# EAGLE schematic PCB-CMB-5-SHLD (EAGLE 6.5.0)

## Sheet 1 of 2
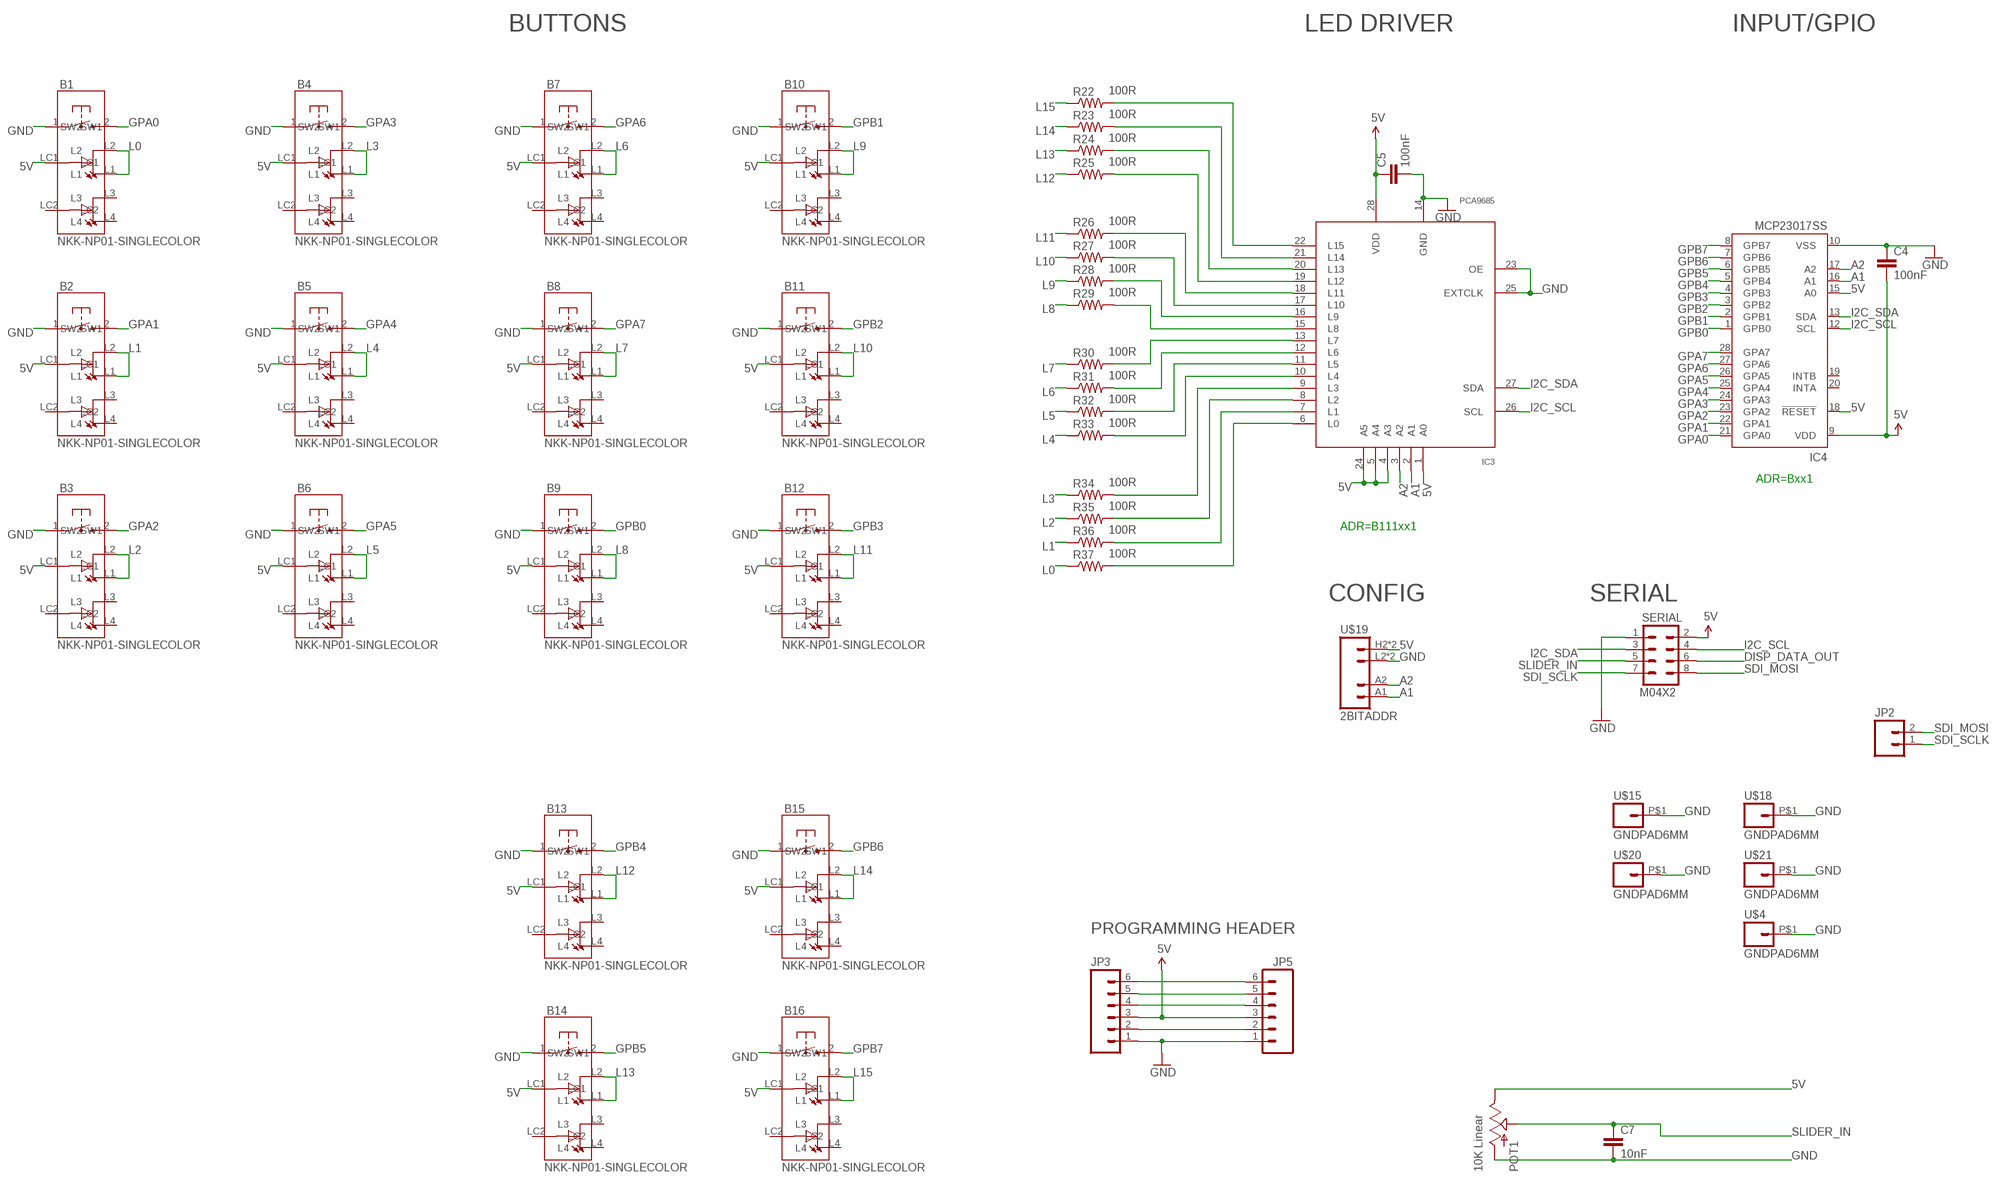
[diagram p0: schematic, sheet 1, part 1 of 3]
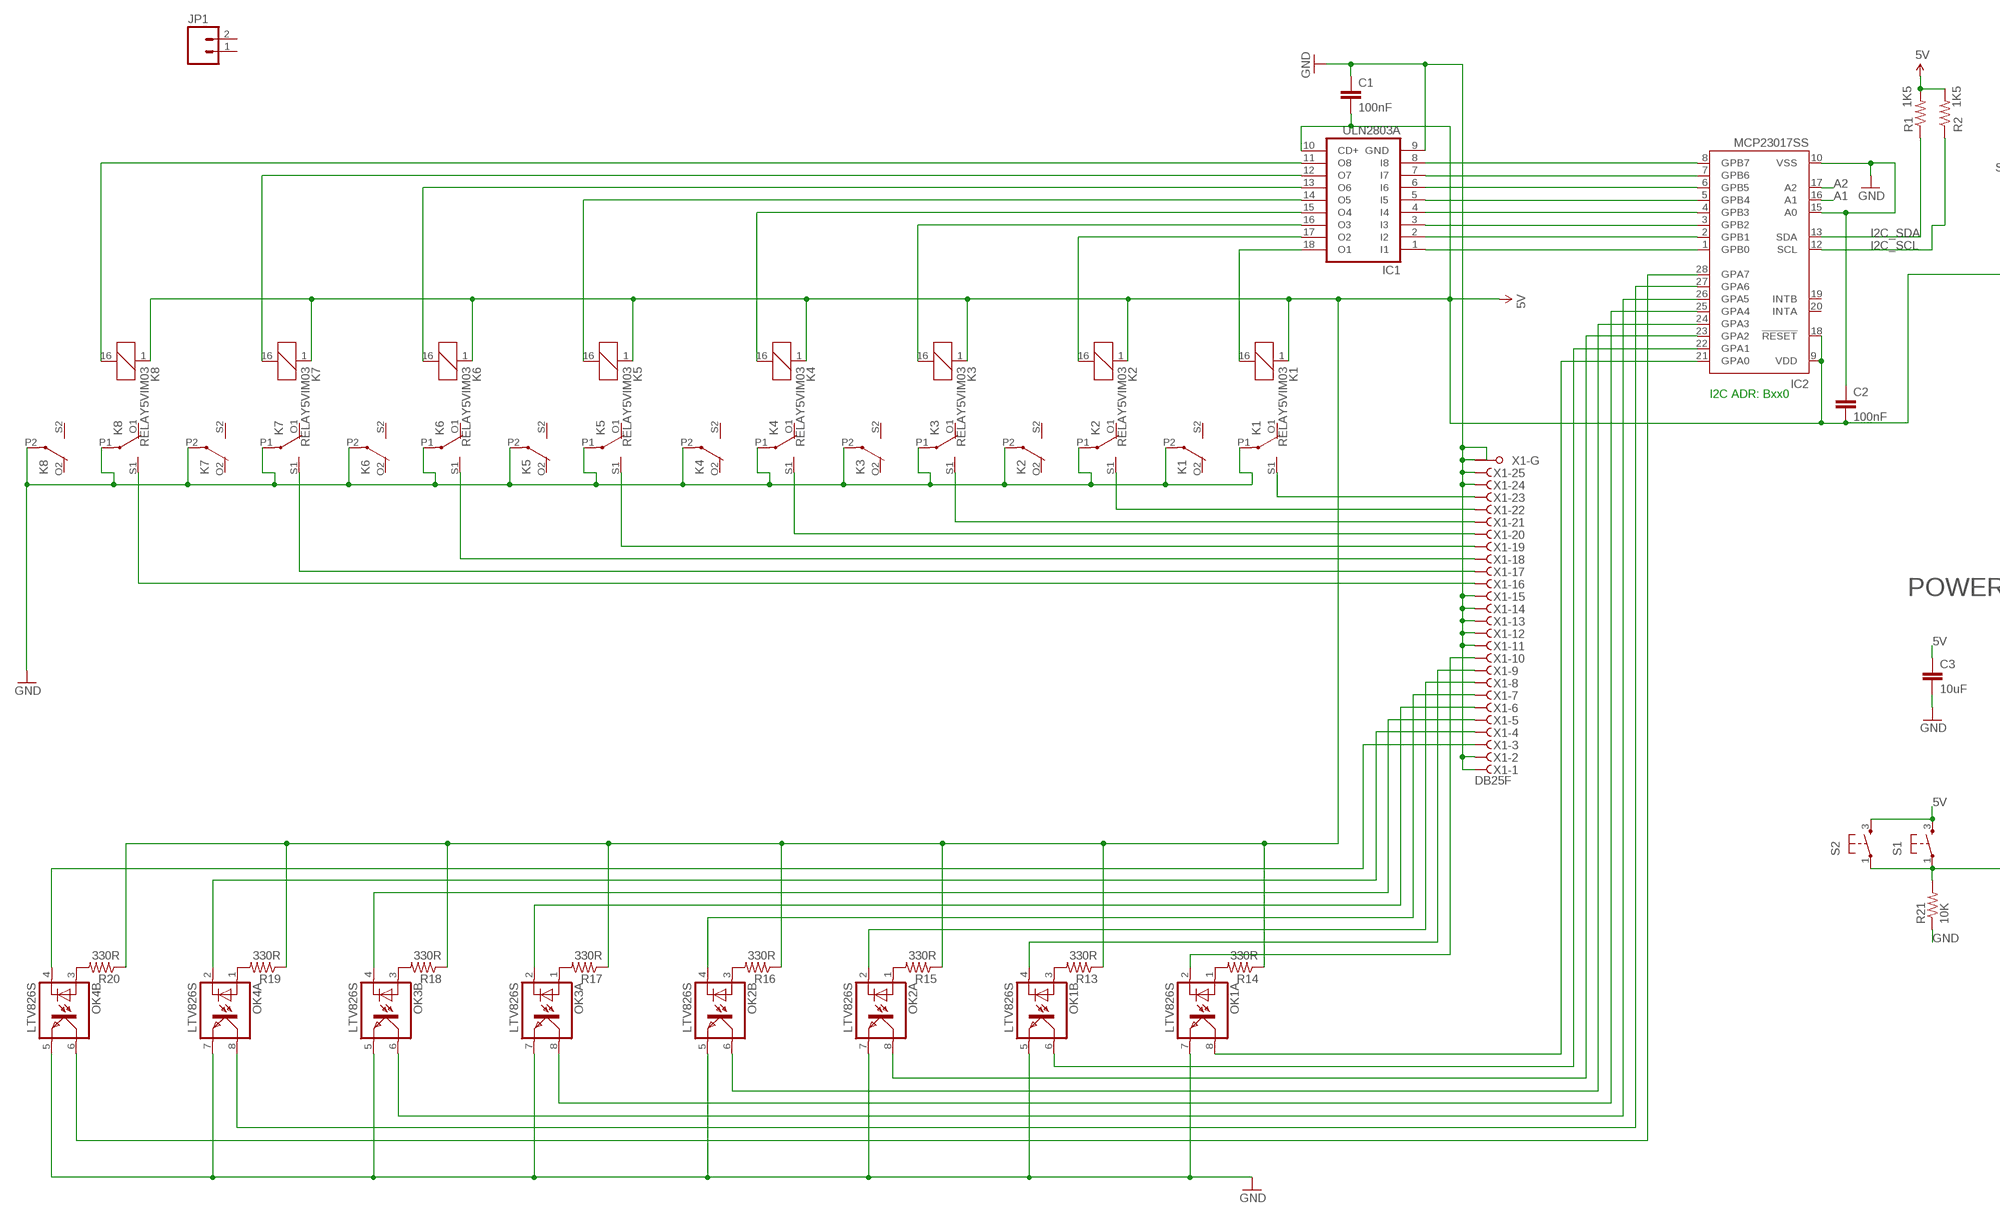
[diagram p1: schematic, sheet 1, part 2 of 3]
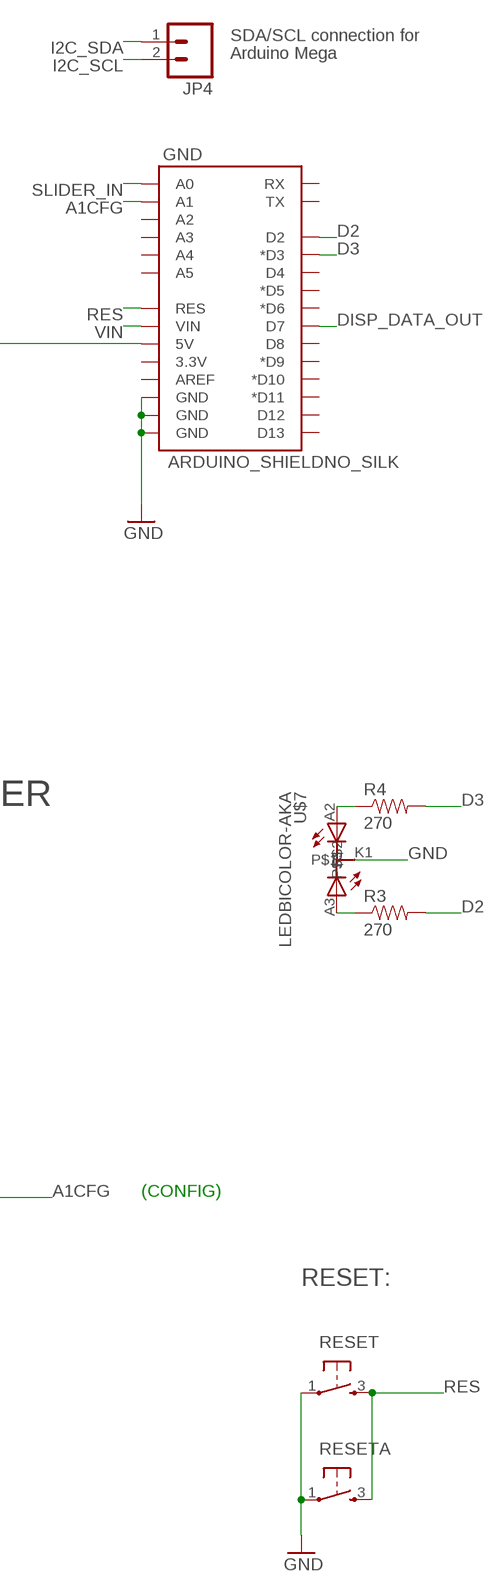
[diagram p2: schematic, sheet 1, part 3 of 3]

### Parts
B1  NKK-NP01-SINGLECOLOR  [NKK-NP01]
B2  NKK-NP01-SINGLECOLOR  [NKK-NP01]
B3  NKK-NP01-SINGLECOLOR  [NKK-NP01]
B4  NKK-NP01-SINGLECOLOR  [NKK-NP01]
B5  NKK-NP01-SINGLECOLOR  [NKK-NP01]
B6  NKK-NP01-SINGLECOLOR  [NKK-NP01]
B7  NKK-NP01-SINGLECOLOR  [NKK-NP01]
B8  NKK-NP01-SINGLECOLOR  [NKK-NP01]
B9  NKK-NP01-SINGLECOLOR  [NKK-NP01]
B10  NKK-NP01-SINGLECOLOR  [NKK-NP01]
B11  NKK-NP01-SINGLECOLOR  [NKK-NP01]
B12  NKK-NP01-SINGLECOLOR  [NKK-NP01]
B13  NKK-NP01-SINGLECOLOR  [NKK-NP01]
B14  NKK-NP01-SINGLECOLOR  [NKK-NP01]
B15  NKK-NP01-SINGLECOLOR  [NKK-NP01]
B16  NKK-NP01-SINGLECOLOR  [NKK-NP01]
C1  100nF  CAP0805  [0805]
C2  100nF  CAP0603-CAP  [0603-CAP]
C3  10uF  CAP0805  [0805]
C4  100nF  CAP0603-CAP  [0603-CAP]
C5  100nF  CAP0603-CAP  [0603-CAP]
C7  10nF  CAP0603-CAP  [0603-CAP]
GND  ARDUINO_SHIELDNO_SILK  [DUEMILANOVE_VIAS]
IC1  ULN2803A  ULN2803ASO18W  [SO18W]
IC2  MCP23017SS  [SSOP28]
IC3  PCA9685  [TSSOP28]
IC4  MCP23017SS  [SSOP28]
JP1  M02PTH  [1X02]
JP2  M02PTH  [1X02]
JP3  M06POLAR  [MOLEX-1X6]
JP4  M02PTH  [1X02]
JP5  M06POLAR  [MOLEX-1X6]
K1  RELAY5VIM03  [DS2Y]
K2  RELAY5VIM03  [DS2Y]
K3  RELAY5VIM03  [DS2Y]
K4  RELAY5VIM03  [DS2Y]
K5  RELAY5VIM03  [DS2Y]
K6  RELAY5VIM03  [DS2Y]
K7  RELAY5VIM03  [DS2Y]
K8  RELAY5VIM03  [DS2Y]
OK1  LTV826S  [DIL8-SMD]
OK2  LTV826S  [DIL8-SMD]
OK3  LTV826S  [DIL8-SMD]
OK4  LTV826S  [DIL8-SMD]
POT1  10K Linear  SLIDER20  [SLIDER20]
R1  1K5  RESISTOR0603-RES  [0603-RES]
R2  1K5  RESISTOR0603-RES  [0603-RES]
R3  270  RESISTOR0603-RES  [0603-RES]
R4  270  RESISTOR0603-RES  [0603-RES]
R13  330R  RESISTOR0603-RES  [0603-RES]
R14  330R  RESISTOR0603-RES  [0603-RES]
R15  330R  RESISTOR0603-RES  [0603-RES]
R16  330R  RESISTOR0603-RES  [0603-RES]
R17  330R  RESISTOR0603-RES  [0603-RES]
R18  330R  RESISTOR0603-RES  [0603-RES]
R19  330R  RESISTOR0603-RES  [0603-RES]
R20  330R  RESISTOR0603-RES  [0603-RES]
R21  10K  RESISTOR0603-RES  [0603-RES]
R22  100R  RESISTOR0603-RES  [0603-RES]
R23  100R  RESISTOR0603-RES  [0603-RES]
R24  100R  RESISTOR0603-RES  [0603-RES]
R25  100R  RESISTOR0603-RES  [0603-RES]
R26  100R  RESISTOR0603-RES  [0603-RES]
R27  100R  RESISTOR0603-RES  [0603-RES]
R28  100R  RESISTOR0603-RES  [0603-RES]
R29  100R  RESISTOR0603-RES  [0603-RES]
R30  100R  RESISTOR0603-RES  [0603-RES]
R31  100R  RESISTOR0603-RES  [0603-RES]
R32  100R  RESISTOR0603-RES  [0603-RES]
R33  100R  RESISTOR0603-RES  [0603-RES]
R34  100R  RESISTOR0603-RES  [0603-RES]
R35  100R  RESISTOR0603-RES  [0603-RES]
R36  100R  RESISTOR0603-RES  [0603-RES]
R37  100R  RESISTOR0603-RES  [0603-RES]
RESET  TAC_SWITCH  [PUSHBUTTON]
RESETA  TAC_SWITCH  [PUSHBUTTON]
S1  TAC_SWITCH  [PUSHBUTTON]
S2  TAC_SWITCH  [PUSHBUTTON]
SERIAL  M04X2  [2X4]
U$4  GNDPAD6MM  [3.2MMPAD6MM]
U$7  LEDBICOLOR-AKA  [LED5MM-BICOLOR]
U$15  GNDPAD6MM  [3.2MMPAD6MM]
U$18  GNDPAD6MM  [3.2MMPAD6MM]
U$19  2BITADDR  [2BITADDR]
U$20  GNDPAD6MM  [3.2MMPAD6MM]
U$21  GNDPAD6MM  [3.2MMPAD6MM]
X1  DB25F  F25HPS  [F25HP]

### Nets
5V [PWR]: B1.LC1 B2.LC1 B3.LC1 B4.LC1 B5.LC1 B6.LC1 B7.LC1 B8.LC1 B9.LC1 B10.LC1 B11.LC1 B12.LC1 B13.LC1 B14.LC1 B15.LC1 B16.LC1 C1.2 C2.2 C3.1 C4.2 C5.1 GND.5V IC1.10(CD+) IC2.9(VDD) IC2.18(!RESET) IC3.1(A0) IC3.4(A3) IC3.5(A4) IC3.24(A5) IC3.28(VDD) IC4.9(VDD) IC4.15(A0) IC4.18(!RESET) JP3.3 JP5.3 K1.1 K2.1 K3.1 K4.1 K5.1 K6.1 K7.1 K8.1 POT1.1(E) R1.2 R2.2 R13.1 R14.1 R15.1 R16.1 R17.1 R18.1 R19.1 R20.1 S1.3 S2.3 SERIAL.2 U$19.H2(VCC) U$19.H3(VCC)
A1: IC2.16(A1) IC3.2(A1) IC4.16(A1) U$19.A1
A1CFG: GND.A1 R21.2 S1.1 S2.1
A2: IC2.17(A2) IC3.3(A2) IC4.17(A2) U$19.A2
D2: GND.D2 R3.2
D3: GND.D3(*D3) R4.2
DISP_DATA_OUT: GND.D7 SERIAL.6
GND [PWR]: B1.1(SW1) B2.1(SW1) B3.1(SW1) B4.1(SW1) B5.1(SW1) B6.1(SW1) B7.1(SW1) B8.1(SW1) B9.1(SW1) B10.1(SW1) B11.1(SW1) B12.1(SW1) B13.1(SW1) B14.1(SW1) B15.1(SW1) B16.1(SW1) C1.1 C2.1 C3.2 C4.1 C5.2 C7.2 GND.GND@0(GND) GND.GND@1(GND) GND.GND@2(GND) IC1.9(GND) IC2.10(VSS) IC2.15(A0) IC3.14(GND) IC3.23(OE) IC3.25(EXTCLK) IC4.10(VSS) JP3.1 JP5.1 K1.P1(2:P) K1.P2(3:P) K2.P1(2:P) K2.P2(3:P) K3.P1(2:P) K3.P2(3:P) K4.P1(2:P) K4.P2(3:P) K5.P1(2:P) K5.P2(3:P) K6.P1(2:P) K6.P2(3:P) K7.P1(2:P) K7.P2(3:P) K8.P1(2:P) K8.P2(3:P) OK1.5(B:EMIT) OK1.7(A:EMIT) OK2.5(B:EMIT) OK2.7(A:EMIT) OK3.5(B:EMIT) OK3.7(A:EMIT) OK4.5(B:EMIT) OK4.7(A:EMIT) POT1.3(A) R21.1 RESET.1 RESETA.1 SERIAL.1 U$4.P$1 U$7.K1 U$15.P$1 U$18.P$1 U$19.L2(GND) U$19.L3(GND) U$20.P$1 U$21.P$1 X1.1(-1:F) X1.2(-2:F) X1.11(-11:F) X1.12(-12:F) X1.13(-13:F) X1.14(-14:F) X1.15(-15:F) X1.24(-24:F) X1.25(-25:F) X1.G1(-G:G1) X1.G2(-G:G2)
GPA0: B1.2(SW2) IC4.21(GPA0)
GPA1: B2.2(SW2) IC4.22(GPA1)
GPA2: B3.2(SW2) IC4.23(GPA2)
GPA3: B4.2(SW2) IC4.24(GPA3)
GPA4: B5.2(SW2) IC4.25(GPA4)
GPA5: B6.2(SW2) IC4.26(GPA5)
GPA6: B7.2(SW2) IC4.27(GPA6)
GPA7: B8.2(SW2) IC4.28(GPA7)
GPB0 [PWR]: B9.2(SW2) IC4.1(GPB0)
GPB1: B10.2(SW2) IC4.2(GPB1)
GPB2: B11.2(SW2) IC4.3(GPB2)
GPB3: B12.2(SW2) IC4.4(GPB3)
GPB4: B13.2(SW2) IC4.5(GPB4)
GPB5: B14.2(SW2) IC4.6(GPB5)
GPB6: B15.2(SW2) IC4.7(GPB6)
GPB7: B16.2(SW2) IC4.8(GPB7)
I2C_SCL: IC2.12(SCL) IC3.26(SCL) IC4.12(SCL) JP4.2 R2.1 SERIAL.4
I2C_SDA: IC2.13(SDA) IC3.27(SDA) IC4.13(SDA) JP4.1 R1.1 SERIAL.3
L0: B1.L1 B1.L2 R37.1
L1: B2.L1 B2.L2 R36.1
L2: B3.L1 B3.L2 R35.1
L3: B4.L1 B4.L2 R34.1
L4: B5.L1 B5.L2 R33.1
L5: B6.L1 B6.L2 R32.1
L6: B7.L1 B7.L2 R31.1
L7: B8.L1 B8.L2 R30.1
L8: B9.L1 B9.L2 R29.1
L9: B10.L1 B10.L2 R28.1
L10: B11.L1 B11.L2 R27.1
L11: B12.L1 B12.L2 R26.1
L12: B13.L1 B13.L2 R25.1
L13: B14.L1 B14.L2 R24.1
L14: B15.L1 B15.L2 R23.1
L15: B16.L1 B16.L2 R22.1
N$1 [RELAY LINES]: K1.S1(2:S) X1.23(-23:F)
N$2: IC3.13(L7) R30.2
N$3: JP3.4 JP5.4
N$4: IC1.18(O1) K1.16
N$5: IC1.1(I1) IC2.1(GPB0)
N$6 [RELAY LINES]: K2.S1(2:S) X1.22(-22:F)
N$7: R4.1 U$7.A2
N$8: JP3.5 JP5.5
N$9: IC1.17(O2) K2.16
N$10 [RELAY LINES]: K3.S1(2:S) X1.21(-21:F)
N$11: R3.1 U$7.A3
N$12: JP3.2 JP5.2
N$13: IC1.16(O3) K3.16
N$14 [RELAY LINES]: K4.S1(2:S) X1.20(-20:F)
N$17: IC1.15(O4) K4.16
N$18 [RELAY LINES]: K5.S1(2:S) X1.19(-19:F)
N$19: IC3.12(L6) R31.2
N$21: IC1.14(O5) K5.16
N$22 [RELAY LINES]: K6.S1(2:S) X1.18(-18:F)
N$23: IC3.11(L5) R32.2
N$25: IC1.13(O6) K6.16
N$26 [RELAY LINES]: K7.S1(2:S) X1.17(-17:F)
N$29: IC1.12(O7) K7.16
N$30 [RELAY LINES]: K8.S1(2:S) X1.16(-16:F)
N$31: IC3.10(L4) R33.2
N$33: IC1.11(O8) K8.16
N$34: IC1.2(I2) IC2.2(GPB1)
N$35: IC1.3(I3) IC2.3(GPB2)
N$36: IC1.4(I4) IC2.4(GPB3)
N$37: IC1.5(I5) IC2.5(GPB4)
N$38: IC1.6(I6) IC2.6(GPB5)
N$39: IC1.7(I7) IC2.7(GPB6)
N$40: IC1.8(I8) IC2.8(GPB7)
N$45: JP3.6 JP5.6
N$47: OK1.3(B:A) R13.2
N$48: OK1.1(A:A) R14.2
N$49 [INput lines]: OK1.2(A:C) X1.10(-10:F)
N$50: OK2.1(A:A) R15.2
N$51: IC2.21(GPA0) OK1.8(A:COL)
N$52: OK2.3(B:A) R16.2
N$53: OK3.1(A:A) R17.2
N$54: OK3.3(B:A) R18.2
N$55 [INput lines]: OK3.2(A:C) X1.6(-6:F)
N$56: OK4.1(A:A) R19.2
N$57: OK4.3(B:A) R20.2
N$58: IC3.9(L3) R34.2
N$59: IC3.8(L2) R35.2
N$60 [INput lines]: OK1.4(B:C) X1.9(-9:F)
N$61 [INput lines]: OK2.2(A:C) X1.8(-8:F)
N$62 [INput lines]: OK2.4(B:C) X1.7(-7:F)
N$63: IC2.28(GPA7) OK4.6(B:COL)
N$64 [INput lines]: OK3.4(B:C) X1.5(-5:F)
N$65 [INput lines]: OK4.2(A:C) X1.4(-4:F)
N$66 [INput lines]: OK4.4(B:C) X1.3(-3:F)
N$67: IC3.7(L1) R36.2
N$68: IC2.22(GPA1) OK1.6(B:COL)
N$69: IC2.23(GPA2) OK2.8(A:COL)
N$70: IC2.24(GPA3) OK2.6(B:COL)
N$71: IC2.25(GPA4) OK3.8(A:COL)
N$72: IC2.26(GPA5) OK3.6(B:COL)
N$73: IC2.27(GPA6) OK4.8(A:COL)
N$74: IC3.6(L0) R37.2
N$75: IC3.15(L8) R29.2
N$76: IC3.16(L9) R28.2
N$77: IC3.17(L10) R27.2
N$78: IC3.18(L11) R26.2
N$79: IC3.19(L12) R25.2
N$80: IC3.20(L13) R24.2
N$81: IC3.21(L14) R23.2
N$82: IC3.22(L15) R22.2
RES: GND.RES RESET.3 RESETA.3
SDI_MOSI: JP2.2 SERIAL.8
SDI_SCLK: JP2.1 SERIAL.7
SLIDER_IN: C7.1 GND.A0 POT1.2A(S) SERIAL.5
VIN: GND.VIN
Unconnected: B1.L3 B1.L4 B1.LC2 B2.L3 B2.L4 B2.LC2 B3.L3 B3.L4 B3.LC2 B4.L3 B4.L4 B4.LC2 B5.L3 B5.L4 B5.LC2 B6.L3 B6.L4 B6.LC2 B7.L3 B7.L4 B7.LC2 B8.L3 B8.L4 B8.LC2 B9.L3 B9.L4 B9.LC2 B10.L3 B10.L4 B10.LC2 B11.L3 B11.L4 B11.LC2 B12.L3 B12.L4 B12.LC2 B13.L3 B13.L4 B13.LC2 B14.L3 B14.L4 B14.LC2 B15.L3 B15.L4 B15.LC2 B16.L3 B16.L4 B16.LC2 GND.3.3V GND.A2 GND.A3 GND.A4 GND.A5 GND.AREF GND.D4 GND.D5(*D5) GND.D6(*D6) GND.D8 GND.D9(*D9) GND.D10(*D10) GND.D11(*D11) GND.D12 GND.D13 GND.RX GND.TX IC2.19(INTB) IC2.20(INTA) IC4.19(INTB) IC4.20(INTA) JP1.1 JP1.2 K1.O1(2:O) K1.O2(3:O) K1.S2(3:S) K2.O1(2:O) K2.O2(3:O) K2.S2(3:S) K3.O1(2:O) K3.O2(3:O) K3.S2(3:S) K4.O1(2:O) K4.O2(3:O) K4.S2(3:S) K5.O1(2:O) K5.O2(3:O) K5.S2(3:S) K6.O1(2:O) K6.O2(3:O) K6.S2(3:S) K7.O1(2:O) K7.O2(3:O) K7.S2(3:S) K8.O1(2:O) K8.O2(3:O) K8.S2(3:S)

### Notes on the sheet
- BUTTONS | LED DRIVER | INPUT/GPIO
- ADR=Bxx1
- ADR=B111xx1
- CONFIG | SERIAL
- PROGRAMMING HEADER
- SDA/SCL connection for
- Arduino Mega
- I2C ADR: Bxx0
- POWER
- (CONFIG)
- RESET:

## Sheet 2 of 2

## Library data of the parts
B1-B16 = SKAARHOJ:NKK-NP01-SINGLECOLOR
C1-C5 C7 = SparkFun:CAP: Capacitor
GND = SparkFun:ARDUINO_SHIELD
IC1 = uln-udn:ULN2803A: DRIVER ARRAY
IC2 IC4 = microchip:MCP23017: http://ww1.microchip.com/downloads/en/DeviceDoc/21952a.pdf Source: http://ww1.microchip.com/downloads/en/DeviceDoc/21952a.pdf; MF: MICROCHIP; MPN: MCP23017-E/SS; OC_FARNELL: 1467674; OC_NEWARK: 31K2960
IC3 = wsmith:PCA9685
JP1 JP2 JP4 = SparkFun:M02: Header 2
JP3 JP5 = SparkFun:M06: Header 6 Standard 6-pin 0.1" header. Use with straight break away headers (SKU : PRT-00116), right angle break away headers (PRT-00553), swiss pins (PRT-00743), machine pins (PRT-00117), and female headers (PRT-00115). Molex polarized connector foot print use with SKU : PRT-08094 with associated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
K1-K8 = SKAARHOJ:RELAY5V: RELAY 2 x switch, AxiCom 150 mW 5V
OK1-OK4 = optocoupler:LTV826: OPTO COUPLER Source: LITEON, LTV816.pdf; OC_FARNELL: unknown; OC_NEWARK: unknown
POT1 = SKAARHOJ:SLIDER
R1-R4 R13-R37 = SparkFun:RESISTOR: Resistor
RESET RESETA S1 S2 = SKAARHOJ:TAC_SWITCH: Momentary Switch
SERIAL = SparkFun:M04X2
U$4 U$15 U$18 U$20 U$21 = SKAARHOJ:GNDPAD
U$7 = SKAARHOJ:LEDBICOLOR-AKA
U$19 = SKAARHOJ:2BITADDR
X1 = con-subd:F25HPS: SUB-D; OC_FARNELL: unknown; OC_NEWARK: unknown

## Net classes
0 default: width 0.203 mm, drill 0.406 mm, clearance 0.203 mm
1 PWR: width 0.406 mm, drill 0.61 mm, clearance 0.203 mm
2 RELAY LINES: width 0.305 mm, clearance 0.203 mm
3 INput lines: clearance 0.203 mm

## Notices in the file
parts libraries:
SparkFun: Licensing: CC v3.0 Share-Alike You are welcome to use this library for commercial purposes.
